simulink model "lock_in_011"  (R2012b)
settings: Solver=FixedStepDiscrete  StartTime=0.0  StopTime=0.5  FixedStep=1e-5  MaxStep=1/(100e3)  RelTol=1e-3
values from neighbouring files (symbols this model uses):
  A = 1000    [lock_in01.m]    (also in lock_in011.m; lock_in02.m; lock_in03.m; feder_masse_1.m = [0 1 0 0;-(k1+k2)/m1,-(c1+c2)/m1, k2/m1,c2/m1)
  ampl_ref = 1    [lock_in01.m]    (also in lock_in011.m; lock_in02.m; lock_in03.m)
  ampl_sig = Usig*sqrt(2)    [lock_in01.m]    (also in lock_in011.m; lock_in02.m; lock_in03.m)
  fref = 10e3    (= 10000)    [lock_in011.m]
  fsig = 10e3    (= 10000)    [lock_in01.m]    (also in lock_in011.m; lock_in02.m; lock_in03.m; diff_filter_1.m = 1)
  h = fir1(nord, 1/L)    [lock_in011.m]    (also in TP_1.m = filter(b, a, [1, zeros(1,1000)]); ode2.m = diff(tspan); ode4.m = diff(tspan); suspension_3.m = spectrum.welch)
  L = 0.001    [boost_up1.m]    (also in buck_boost1.m; buck_boost2.m; buck_down1.m; buck_down2.m)
  phase_ref = 0    [lock_in01.m]    (also in lock_in011.m; lock_in02.m; lock_in03.m)
  phase_sig = 0    [lock_in01.m]    (also in lock_in011.m; lock_in02.m; lock_in03.m)
  Ts = 1e-5    (= 1e-05)    [lock_in01.m]    (also in lock_in011.m; lock_in02.m; lock_in03.m)
  v_rausch = (rausch_effektiv)^2*fs    (= 2.5e-12)    [lock_in01.m]    (also in lock_in011.m; lock_in02.m; lock_in03.m)
undefined symbols (not defined in the file or in its folder): dBW, Fs, get, Hertz, sided, Two
libraries: dspsnks4 x2, dspsigops x1, dspstat3 x1

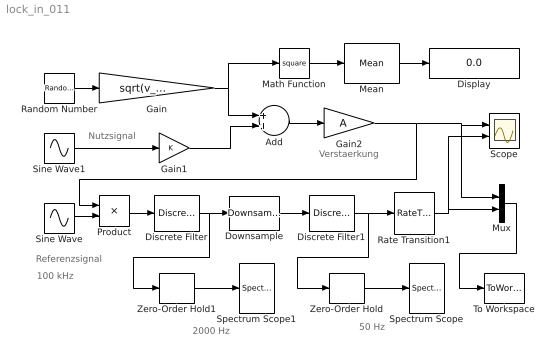
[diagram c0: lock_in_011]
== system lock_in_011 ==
  note: 100 kHz
  note: 50 Hz
  note: 2000 Hz
  note: Verstaerkung
  note: Referenzsignal
  note: Nutzsignal
  Add : Sum
  Discrete Filter : DiscreteFilter  Numerator=[h]  Denominator=[1]  SampleTime=Ts
  Discrete Filter1 : DiscreteFilter  Numerator=[h]  Denominator=[1]  SampleTime=Ts*100
  Display : Display
  Downsample : dspsigops/Downsample  N=L  phase=0  RateOptions=Allow multirate processing  smode=Force single rate  fmode=Maintain input frame size  ic=0
  Gain : Gain  Gain=sqrt(v_rausch)
  Gain1 : Gain
  Gain2 : Gain  Gain=A
  Math Function : Math  Operator=square
  Mean : dspstat3/Mean  run=on  reset_popup=None  InputProcessing=Columns as channels (frame based)  directionMode=Each column  dimension=1  treatSBRowAsCol=on  roiEnable=off  roiType=Rectangles  roiPortion=Entire ROI  roiOutput=Individual statistics for each ROI  roiFlag=off  outputDataTypeStr=Inherit: Same as accumulator  outputLastDataTypeStr=Inherit: Same as accumulator  outputMin=[]  outputMax=[]  roundingMode=Floor  overflowMode=off
  Mux : Mux  Inputs=2
  Product : Product
  Random Number : RandomNumber  SampleTime=Ts
  Rate Transition1 : RateTransition  OutPortSampleTime=Ts
  Scope : Scope  NumInputPorts=2
  Sine Wave : Sin  Amplitude=ampl_ref  Frequency=2*pi*fref  Phase=phase_ref  SampleTime=Ts
  Sine Wave1 : Sin  Amplitude=ampl_sig  Frequency=2*pi*fsig  Phase=phase_sig  SampleTime=Ts
  Spectrum Scope : dspsnks4/Spectrum Scope  ScopeProperties=on  Domain=Frequency  HorizSpan=1  UseBuffer=on  BufferSize=256  Overlap=0  TreatMby1Signals=One channel  inpFftLenInherit=on  FFTlength=256  numAvg=1  DisplayProperties=off  AxisGrid=on  Memory=off  FrameNumber=on  AxisLegend=off  AxisZoom=off  OpenScopeAtSimStart=on  OpenScopeImmediately=off  FigPos=get(0,'defaultfigureposition')  AxisProperties=off  XUnits=Hertz  XRange=Two-sided ((-Fs/2...Fs/2])  XDisplay=0  InheritXIncr=on  XIncr=0.02  XLabel=Samples  XLimit=User-defined  YUnits=dBW/Hertz  XMax=25  XMin=-25  YLabel=Magnitude-squared, dB  LineProperties=off  wintypeSpecScope=Hamming  RsSpecScope=50  betaSpecScope=5  winsampSpecScope=Periodic  XAxisParamsVer=6.9  isFrameUpgraded=on
  Spectrum Scope1 : dspsnks4/Spectrum Scope  ScopeProperties=on  Domain=Frequency  HorizSpan=1  UseBuffer=on  BufferSize=256  Overlap=0  TreatMby1Signals=One channel  inpFftLenInherit=on  FFTlength=256  numAvg=10  DisplayProperties=off  AxisGrid=on  Memory=off  FrameNumber=on  AxisLegend=off  AxisZoom=off  OpenScopeAtSimStart=on  OpenScopeImmediately=off  FigPos=get(0,'defaultfigureposition')  AxisProperties=off  XUnits=Hertz  XRange=Two-sided ((-Fs/2...Fs/2])  XDisplay=0  InheritXIncr=on  XIncr=0.02  XLabel=Samples  XLimit=User-defined  YUnits=dBW/Hertz  XMax=1000  XMin=-1000  YLabel=Magnitude-squared, dB  LineProperties=off  wintypeSpecScope=Hamming  RsSpecScope=50  betaSpecScope=5  winsampSpecScope=Periodic  XAxisParamsVer=6.9  isFrameUpgraded=on
  To Workspace : ToWorkspace  VariableName=y  SampleTime=-1  SaveFormat=Structure With Time
  Zero-Order Hold : ZeroOrderHold  SampleTime=1/50
  Zero-Order Hold1 : ZeroOrderHold  SampleTime=1/2000
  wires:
  Sine Wave/1 -> Product/2
  Random Number/1 -> Gain/1
  Sine Wave1/1 -> Gain1/1
  Gain1/1 -> Add/2
  Gain/1 -> Add/1, Math Function/1
  Add/1 -> Gain2/1
  Product/1 -> Discrete Filter/1
  Math Function/1 -> Mean/1
  Mean/1 -> Display/1
  Mux/1 -> To Workspace/1
  Downsample/1 -> Discrete Filter1/1
  Gain2/1 -> Product/1, Mux/1, Scope/1
  Rate Transition1/1 -> Mux/2, Scope/2
  Zero-Order Hold/1 -> Spectrum Scope/1
  Discrete Filter1/1 -> Zero-Order Hold/1, Rate Transition1/1
  Zero-Order Hold1/1 -> Spectrum Scope1/1
  Discrete Filter/1 -> Zero-Order Hold1/1, Downsample/1
